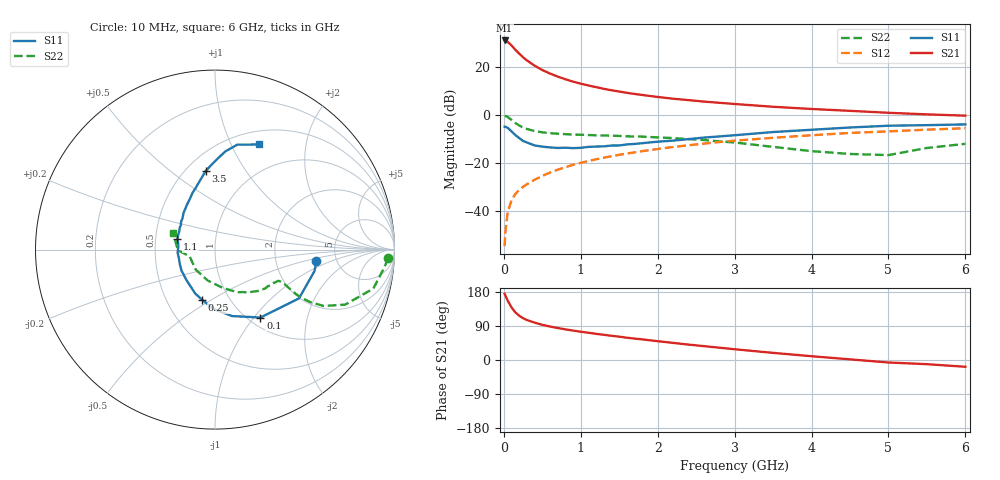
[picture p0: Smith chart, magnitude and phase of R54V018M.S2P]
! SIEMENS Small Signal Semiconductors
! BFR183
! Si NPN RF Bipolar Junction Transistor in SOT23
! VCE = 4 V  IC = 18 mA
! Common Emitter S-Parameters:  May  1996
# GHz  S  MA  R  50
!  f  S11  S21  S12  S22
! GHz  MAG  ANG  MAG  ANG  MAG  ANG  MAG  ANG
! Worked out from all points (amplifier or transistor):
!   36 points, 10 MHz to 6 GHz, reference 50 ohm
!   highest |S21| = 30.9 dB at 10 MHz (marker M1)
!   |S21| within 3 dB of that: start of sweep to 125.6 MHz
!   unconditionally stable (mu >= 1): 597.1 MHz to 2.4 GHz
!   at 250 MHz: K = 0.78, MSG = 26.9 dB, |S12| = -29.8 dB
!   at 1.4 GHz: K = 1.04, MAG = 12.4 dB, |S12| = -17.1 dB
!   at 6 GHz: K = 0.90, MSG = 2.6 dB, |S12| = -5.5 dB
!   S11 on the Smith chart (normalised r, x): 10 MHz: 3.51, -0.66; 100 MHz: 1.13, -1.08; 250 MHz: 0.75, -0.46; 1.1 GHz: 0.65, +0.08; 3.5 GHz: 0.62, +0.68; 6 GHz: 0.65, +1.29
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0.01  0.5689 -6.4  35.05 174.8  0.0019 86.5  0.9651 -2.8
0.02  0.5671 -12.2  34.54 170.0  0.0038 85.4  0.9505 -5.7
0.05  0.5411 -30.2  32.78 156.7  0.0096 78.0  0.9089 -13.8
0.1  0.4554 -56.2  27.58 138.8  0.017 71.1  0.7877 -22.9
0.15  0.3826 -75.5  22.43 125.7  0.023 68.1  0.6824 -27.4
0.2  0.3315 -91.3  18.67 116.8  0.0278 67.2  0.6052 -28.9
0.25  0.2884 -104.4  15.7 110.4  0.0324 67.6  0.5477 -29.1
0.3  0.2683 -114.3  13.52 105.5  0.0365 68.4  0.5109 -28.7
0.4  0.2332 -132.7  10.52 98.6  0.0454 69.5  0.4645 -27.5
0.5  0.2204 -147.8  8.533 92.8  0.0545 70.3  0.4358 -26.5
0.6  0.212 -157.6  7.217 88.3  0.0638 70.5  0.4188 -26.0
0.7  0.2066 -167.7  6.253 84.4  0.0731 70.8  0.4081 -25.9
0.8  0.2093 -175.4  5.493 80.9  0.0824 70.4  0.3995 -26.1
0.9  0.205 176.6  4.907 77.6  0.0923 69.9  0.3921 -26.4
1.1  0.2174 164.1  4.087 71.9  0.1108 69.0  0.3833 -28.3
1.3  0.2232 153.2  3.481 66.5  0.1301 67.4  0.3739 -30.2
1.6  0.2448 140.4  2.873 58.8  0.1587 64.8  0.3605 -34.2
2.2  0.2937 122.3  2.17 45.2  0.2162 58.7  0.3318 -44.1
3.5  0.4423 96.6  1.478 18.8  0.3358 42.6  0.2175 -78.6
4.5  0.5492 84.1  1.216 1.7  0.4233 30.1  0.1551 -133.3
5.5  0.6142 72.2  1.028 -11.0  0.4956 18.4  0.2067 -178.9
6  0.6368 67.1  0.967 -17.9  0.5302 10.8  0.2518 158.1
